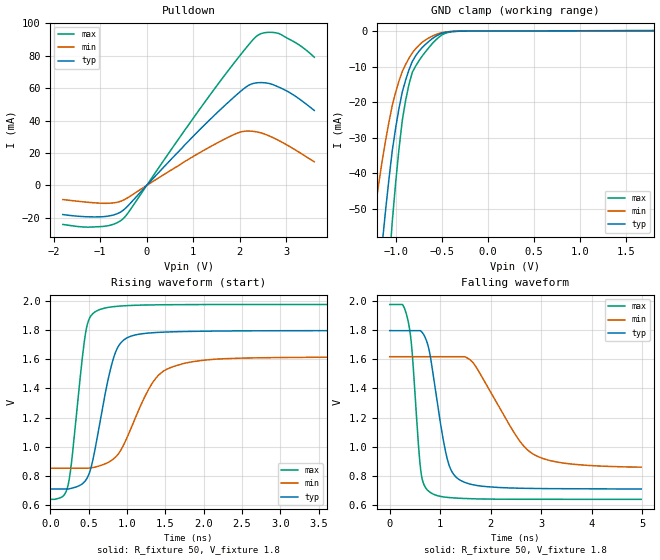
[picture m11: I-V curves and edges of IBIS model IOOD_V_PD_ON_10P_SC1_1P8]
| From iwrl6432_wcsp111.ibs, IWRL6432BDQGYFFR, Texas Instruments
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|   Model Cell IOOD_V_PD_ON_10P_SC1_1P8
|IOOD_V_PD_ON_10P_SC1_1P8
[Model]   IOOD_V_PD_ON_10P_SC1_1P8
Model_type   I/O_open_drain
Polarity   Non-Inverting
Enable   Active-Low
Vinl =  0.63
Vinh =  1.17
Cref =  15pF
Rref =  100.0000M
Vref =  0V
Vmeas =  0.9
|   typ   min   max
C_comp   2.290246p   2.205796p   2.292736p
[Model Spec]
Vinl   0.63   0.567   0.693
Vinh   1.17   1.053   1.287
[Temperature Range]   25   125   -40
[Voltage Range]   1.8   1.62   1.98
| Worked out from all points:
|   slope of the pulldown table from 0 to 0.27 V, typ, clamps not added: 32.2 ohm
|   GND clamp passes 1 mA (typ) near -0.53 V on its own axis
|   rising waveform, R_fixture 50, V_fixture 1.8: 20-80 % time 246ps typ, 417ps min, 160ps max; typ from 0.708 V to 1.8 V
|   falling waveform, R_fixture 50, V_fixture 1.8: 20-80 % time 308ps typ, 788ps min, 165ps max; typ from 1.8 V to 0.708 V
| Where Nom  PVT is Nominal Process, 1.8V, 25C
|   Fast PVT is Strong Process,  1.98V, -40C
|   Slow PVT is Weak Process,   1.62V, 125C
[Pulldown]
|   voltage   I(typ)   I(min)   I(max)
-1.8V     -17.92mA   -8.674mA   -24.03mA
-927.3mV  -19.22mA   -10.99mA   -25.2mA
-654.5mV  -17.65mA   -10.46mA   -23.22mA
-490.9mV  -14.97mA   -8.904mA   -20.12mA
818.2mV   25.05mA    14.78mA    34.16mA
1.691V    49.7mA     28.87mA    68.58mA
2.127V    60.63mA    33.53mA    84.59mA
2.4V      63.43mA    32.85mA    92.9mA
2.618V    62.99mA    30.74mA    94.47mA
2.836V    60.69mA    27.76mA    93.76mA
3.273V    53.49mA    20.53mA    86.73mA
3.6V      46.26mA    14.64mA    79.12mA
[GND_clamp]
|   voltage   I(typ)   I(min)   I(max)
-1.8V     -270.2mA   -170.2mA   -430.1mA
-1.255V   -91.66mA   -55.91mA   -148.4mA
-1.145V   -59.91mA   -36.45mA   -97.1mA
-1.109V   -50.48mA   -30.83mA   -81.56mA
-1.073V   -41.73mA   -25.65mA   -67.06mA
-1.036V   -33.67mA   -20.93mA   -53.6mA
-927.3mV  -17.08mA   -11.35mA   -25.06mA
-854.5mV  -10.88mA   -7.623mA   -14.95mA
-781.8mV  -6.944mA   -4.955mA   -9.81mA
-636.4mV  -2.852mA   -1.883mA   -4.568mA
-381.8mV  -107.5uA   -91.83uA   -158.4uA
1.8V      101.9uA    59.86uA    152.6uA
[Ramp]
| variable   typ   min   max
dV/dt_f 0.66096346/0.31032052n 0.46741953/0.81005029n 0.81000902/0.16620273n
dV/dt_r  0.6586759/0.43206812n 0.47399668/1.0503576n 0.81471515/0.23033778n
R_load = 50
[Rising Waveform]
R_fixture = 50
V_fixture = 1.8
V_fixture_min = 1.62
V_fixture_max = 1.98
|   time   V(typ)   V(min)   V(max)
0s        708.4mV    851.3mV    637.9mV
228.2ps   708.4mV    851.3mV    727.1mV
277.2ps   714.2mV    851.3mV    893.6mV
460ps     767.5mV    851.3mV    1.782V
607.4ps   1.051V     862.8mV    1.934V
832.2ps   1.622V     919.4mV    1.963V
1.059ns   1.761V     1.135V     1.971V
1.376ns   1.785V     1.471V     1.975V
1.754ns   1.792V     1.574V     1.977V
4.974ns   1.798V     1.617V     1.977V
[Falling Waveform]
R_fixture = 50
V_fixture = 1.8
V_fixture_min = 1.62
V_fixture_max = 1.98
|   time   V(typ)   V(min)   V(max)
0s        1.798V     1.619V     1.978V
367.8ps   1.798V     1.619V     1.858V
439.5ps   1.798V     1.619V     1.666V
613.8ps   1.796V     1.619V     836.4mV
784.1ps   1.656V     1.619V     689mV
1.123ns   936.1mV    1.619V     651.2mV
1.374ns   773.1mV    1.619V     644.4mV
1.662ns   736.2mV    1.571V     640.6mV
2.825ns   711.9mV    951.4mV    637.2mV
4.974ns   708.1mV    858.5mV    637mV
